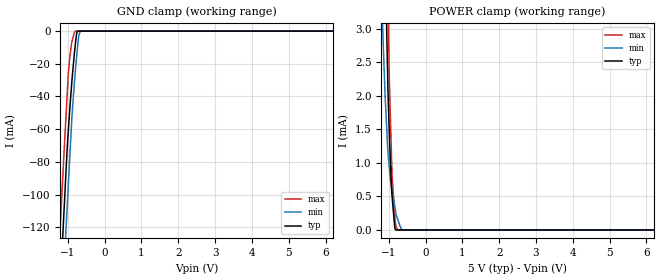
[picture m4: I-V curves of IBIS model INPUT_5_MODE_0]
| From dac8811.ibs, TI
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|   Input INPUT_MODE 5V Model
[Model] INPUT_5_MODE_0
Model_type Input
| Signals   SDI(2)
Vinl = 0.8
Vinh = 2.4
|   typ   min   max
|   (nom PVT)   (Fast PVT)   (slow PVT)
C_comp   9.321e-13   9.257e-13   9.549e-13
| Where   nom PVT is  Nominal Process, 5.0V, 26C
|   Fast PVT is Strong Process, 5.5V, -40C
|   Slow PVT is Weak Process, 4.5V, 86C
[Voltage Range]   5   4.5   5.5
|Ambient Temperature   25   85   -40
|Junction Temperature
[Temperature Range]   26   86   -40
[Power Clamp Reference]   5   4.5   5.5
[GND Clamp Reference]   0   0   0
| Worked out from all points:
|   GND clamp passes 1 mA (typ) near -0.75 V on its own axis
|   POWER clamp passes 1 mA (typ) near -0.95 V on its own axis
[GND Clamp]
|   Voltage   I(typ)   I(min)   I(max)
-5V       -2.042A    -2.07A     -2.017A
-1.21V    -158.7mA   -194.5mA   -122.3mA
-1.153V   -132.5mA   -167.6mA   -96.19mA
-1.115V   -115.3mA   -150.9mA   -79.84mA
-1.079V   -99.07mA   -134.6mA   -63.99mA
-1.022V   -73.9mA    -109.5mA   -40.7mA
-941mV    -46.05mA   -74.67mA   -15.06mA
-887mV    -29.92mA   -51.99mA   -6.371mA
-790mV    -7.015mA   -23.11mA   0A
-707mV    0A         -3.813mA   0A
-662mV    0A         0A         0A
10V       0A         0A         0A
[POWER Clamp]
|   Voltage   I(typ)   I(min)   I(max)
-5V       164.4mA    136.5mA    204.1mA
-1.161V   5.956mA    3.003mA    9.27mA
-1.099V   4.17mA     2.02mA     6.677mA
-1.056V   3.055mA    1.547mA    4.949mA
-1.015V   1.991mA    1.128mA    3.399mA
-975mV    1.305mA    879.7uA    2.091mA
-925mV    650.3uA    653.5uA    1.128mA
-902.5mV  466.7uA    578.2uA    762.5uA
-835mV    37.15uA    352.2uA    233.3uA
-797mV    0A         225uA      47.92uA
-639.5mV  0A         0A         0A
10V       0A         0A         0A
